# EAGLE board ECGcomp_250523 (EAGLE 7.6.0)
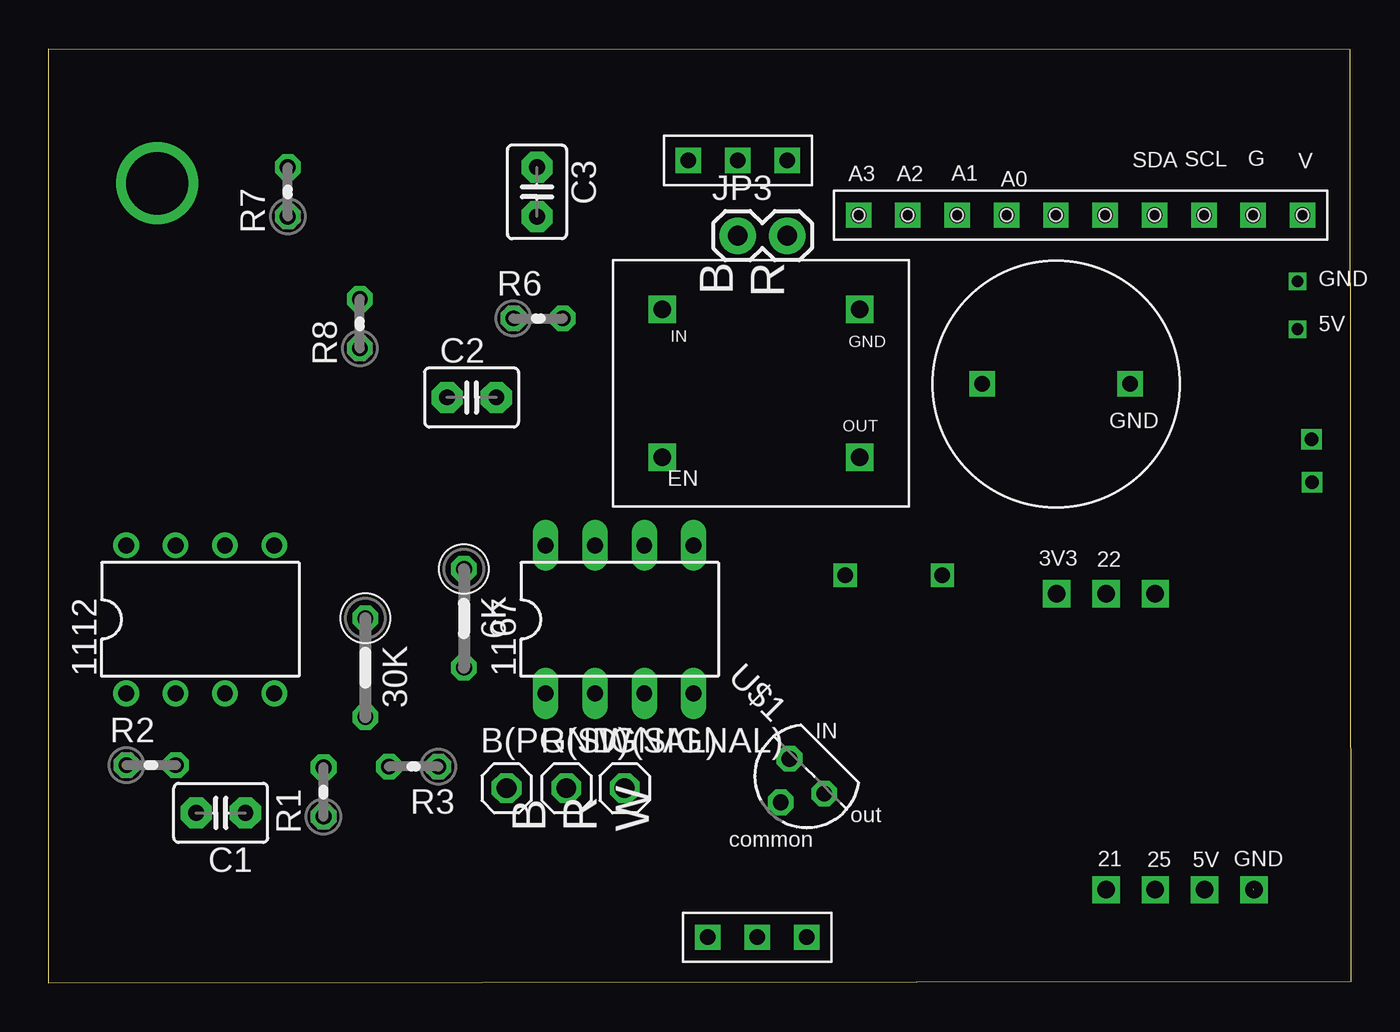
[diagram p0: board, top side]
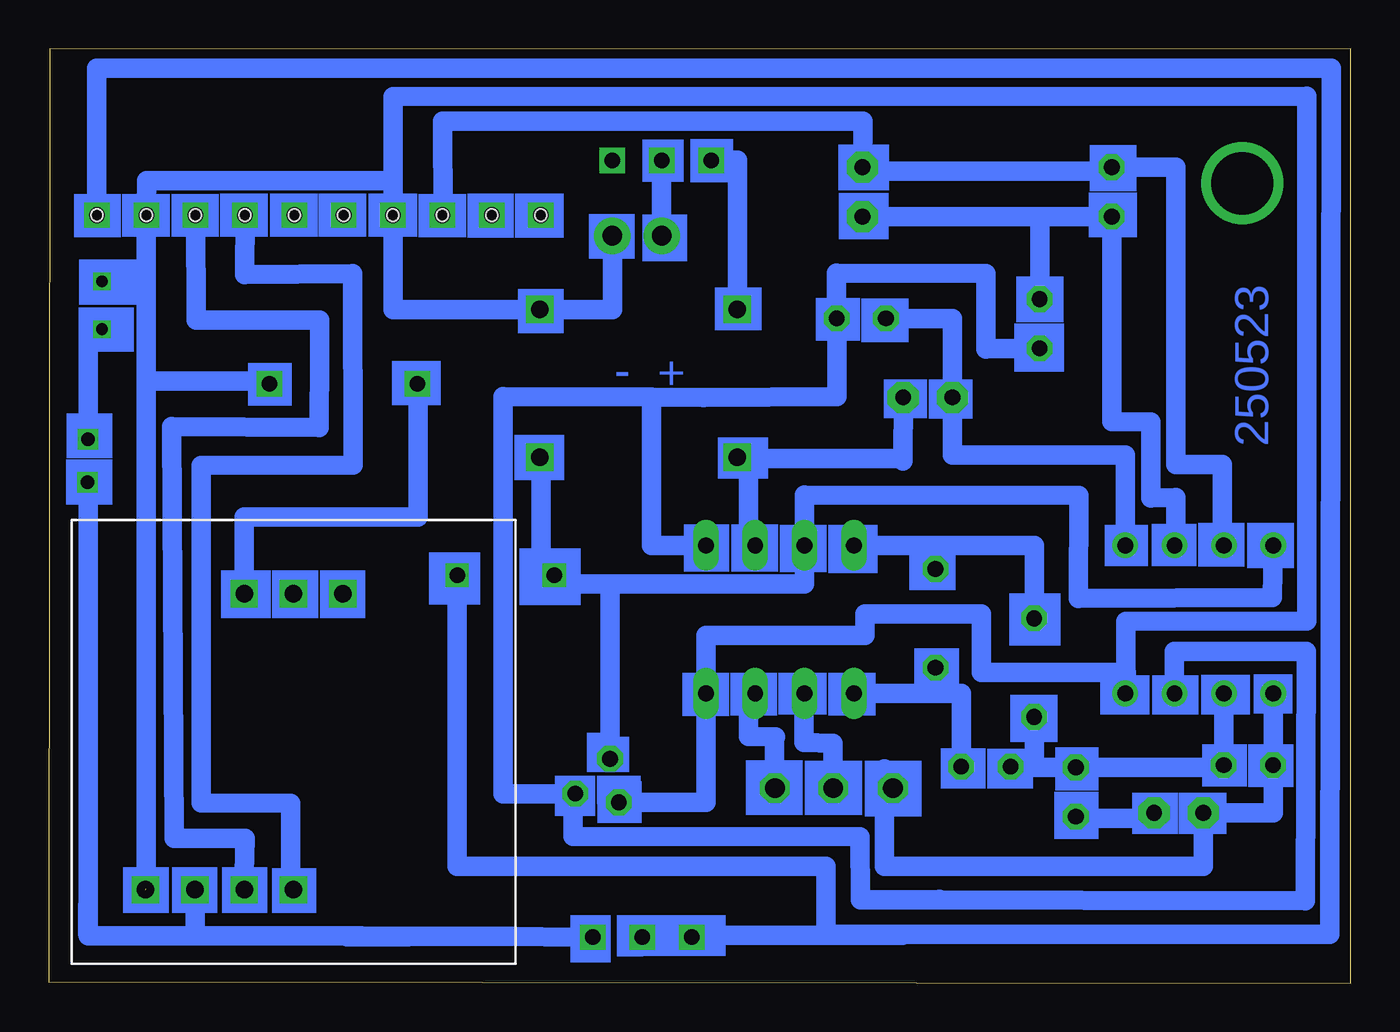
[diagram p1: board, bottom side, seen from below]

Size 67.03 x 48.1 mm. Coordinates in mm from the lower left corner, seen from the top.
Outline: 66.98,48.08 67.03,0.08 0,0 0,48.1 66.98,48.08
Copper layers (1*16): Top 0.035mm / dielectric 1.5mm / Bottom 0.035mm
Design rules "Fusion_eagle_rule_v1.1": minimum track width 6mil, minimum drill 12mil, track to track 6mil, track to pad 6mil, pad to pad 6mil, via to via 6mil, smd to smd 0mil, copper to edge 10mil, drill to drill 10mil, minimum pad ring 10mil, minimum via ring 6mil, stop-mask expansion 2mil, vias tented up to drill 100mil, thermal gap 10mil
Net classes: 0 default: width 1.016 mm

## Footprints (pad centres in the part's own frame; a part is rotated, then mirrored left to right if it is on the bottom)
0207/5V = drill 0.813 octagon: 1 -2.54,0; 2 2.54,0
DIL08 = drill 0.813 pad 1.27: 1 -3.81,-3.81; 2 -1.27,-3.81; 3 1.27,-3.81; 4 3.81,-3.81; 5 3.81,3.81; 6 1.27,3.81; 7 -1.27,3.81; 8 -3.81,3.81
DIL08' = drill 0.813 long: 1 -3.81,-3.81; 2 -1.27,-3.81; 3 1.27,-3.81; 4 3.81,-3.81; 5 3.81,3.81; 6 1.27,3.81; 7 -1.27,3.81; 8 -3.81,3.81
1X01 = drill 1.016 octagon: 1 0,0
C2.5-3 = drill 0.813 pad 1.6 octagon: 1 -1.27,0; 2 1.27,0
1X02 = drill 1.016 pad 1.88: 1 0,0; 2 2.54,0
0204V = drill 0.813 octagon: 1 -1.27,0; 2 1.27,0
TO226AA = drill 0.813 octagon: 1 -1.27,0; 2 0,1.905; 3 1.27,0
2 = drill 0.9 square: 3V3 -5.08,0; 5V 10.16,-7.62; G 10.16,-10.16; G19 -5.08,-5.08; G21 10.16,-2.54; G22 -5.08,-2.54; G25 10.16,-5.08
BUZZER = drill 0.8 square: LONG+ 2.54,0; SHORT- -5.08,0
SW1 = drill 0.8 square: SW1 -2.54,1.27; SW2 -5.08,1.27; SW3 -7.62,1.27
ADCHENGE2 = drill 0.8 square: 5V 7.62,5.08; A0 -7.62,5.08; A1 -10.16,5.08; A2 -12.7,5.08; A3 -15.24,5.08; ADDR -2.54,5.08; ALERT -5.08,5.08; GND 5.08,5.08; SCL 2.54,5.08; SDA 0,5.08 | hole 0.6: -15.24,5.08; -12.7,5.08; -10.16,5.08; 7.62,5.08; 5.08,5.08; 2.54,5.08; 0,5.08; -2.54,5.08; -5.08,5.08; -7.62,5.08
MCP1640 = drill 0.9 square: EN 2.54,-5.08; GND -5.08,5.08; VIN -5.08,-5.08; VOUT 2.54,5.08

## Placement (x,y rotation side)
6K  R5  [0207/5V]  21.37,18.78 270 top
30K  R4  [0207/5V]  16.29,16.24 270 top
1112  LT1112  [DIL08]  7.79,18.73 0 top
1167  LT1167CN8  [DIL08']  29.38,18.73 0 top
B(PGND)  [1X01]  23.56,10.03 0 top
C1  0.01uF  [C2.5-3]  8.85,8.76 180 top
C2  0.47uF  [C2.5-3]  21.76,30.16 0 top
C3  15nF  [C2.5-3]  25.13,40.74 270 top
JP3  Battery  [1X02]  35.47,38.48 0 top
R1  12k  [0204V]  14.14,9.84 90 top
R2  1M  [0204V]  5.26,11.22 0 top
R3  30k  [0204V]  18.78,11.15 180 top
R6  6k  [0204V]  25.19,34.22 0 top
R7  10k  [0204V]  12.3,40.74 90 top
R8  100k  [0204V]  16.01,33.95 90 top
R(SIGNAL)  [1X01]  26.64,10.03 0 top
U$1  TLE2426CLP  [TO226AA]  39.02,10.65 135 top
U$2  2  [2]  51.88,14.96 270 bottom
U$3  BUZZER  [BUZZER]  50.58,30.84 180 top
U$4  SW1  [SW1]  31.39,3.63 180 top
U$5  ADCHENGE2  [ADCHENGE2]  56.92,34.46 0 top
U$6  SW1  [SW1]  30.39,43.63 180 top
U$8  MCP1640  [MCP1640]  36.66,29.61 270 top
W(SIGNAL)  [1X01]  29.64,10.03 0 top

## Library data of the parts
6K 30K R1-R3 R6-R8 = resistor
1112 = linear
1167 = linear-technology; MPN: LT1168CN8#PBF; OC_FARNELL: 1330587; OC_NEWARK: 57M2327
B(PGND) R(SIGNAL) W(SIGNAL) = pinhead
C1-C3 = capacitor-wima
JP3 = SparkFun-Connectors
U$1 = tle2426
U$2 = M5Atom_Lite
U$3 = buzzer
U$4 U$6 = Switch1
U$5 = ADChenge
U$8 = MCP1640

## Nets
B1: 1112.3 1167.5 R6.2 R8.1 U$1.1
N$1: 1112.1 B(PGND).1 C1.2 R2.1
N$2: W(SIGNAL).1
N$3: 30K.2 1112.2 R1.2 R2.2 R3.2
N$4: 6K.2 1167.1 R3.1
N$5: 6K.1 30K.1 1167.8
N$6: 1167.2 R(SIGNAL).1
N$7: 1112.8 1167.7 U$1.3 U$8.VOUT
N$8: 1167.6 C2.2
N$9: 1112.5 C2.1 R6.1
N$10: 1112.6 C3.2 R7.1 R8.2
N$11: C1.1 R1.1
N$12: 1112.7 C3.1 R7.2 U$5.A1
N$13: 1112.4 1167.4 JP3.2 U$1.2 U$5.A0 U$8.GND
N$16: JP3.1 U$6.SW2
N$17: U$5.5V
N$18: U$2.G U$3.SHORT- U$5.GND
N$19: U$2.G25 U$5.SCL
N$20: U$2.G21 U$5.SDA
N$21: U$2.G19 U$3.LONG+
N$22: U$6.SW1 U$8.VIN
S$2: U$2.5V

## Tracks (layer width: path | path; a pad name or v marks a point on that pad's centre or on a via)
B1
  Bottom 1.016: 1112.3 9.08,14.92 9.08,17.08 2.29,17.08 2.34,4.24 25.24,4.29 | 40.01,9.66 U$1.1 | 18.78,32.68 18.78,36.53 26.46,36.56 R6.2 26.58,34.2 26.45,34.2 26.45,30.21 33.32,30.16 36,30.17 | U$1.1 43.65,9.75 43.65,30.21 36,30.17 | 36,30.17 36,22.54 1167.5 | R8.1 18.78,32.68 | 18.78,32.68 18.78,32.65 | U$1.1 40,9.75 40.02,7.56 25.27,7.53 25.24,4.29 | 25.24,4.29 21.18,4.31
N$1
  Bottom 1.016: 1112.1 3.99,14.92 R2.1 3.99,8.76 C1.2 7.58,6 24,6 24,11.03 B(PGND).1
N$2
  Bottom 1.016: 29.67,12.51 W(SIGNAL).1
N$3
  Bottom 1.016: 1112.2 6.53,14.92 R2.2 6.53,11.11 R1.2 16.29,11.11 | 16.29,11.11 17.51,11.11 R3.2 | 30K.2 16.29,11.11
N$4
  Bottom 1.016: 1167.1 25.41,14.92 21.37,14.92 | 21.37,14.92 20.05,14.92 R3.1 | 6K.2 21.37,14.92
N$5
  Bottom 1.016: 1167.8 21.37,22.54 | 21.37,22.54 16.29,22.54 30K.1 | 6K.1 21.37,22.54
N$6
  Bottom 1.016: 1167.2 28.15,14.92 28.15,12.38 26.64,12.34 R(SIGNAL).1
N$7
  Bottom 1.016: 1112.8 4.02,19.85 14.03,19.8 13.98,25.11 28.11,25.13 1167.7 28.11,20.56 38.12,20.56 | 38.12,20.56 U$1.3 | 38.12,20.56 41.69,20.56 41.69,27.07 U$8.VOUT
N$8
  Bottom 1.016: C2.2 23.05,26.88 23.05,27 31,27 31,22.54 1167.6
N$9
  Bottom 1.016: R6.1 20.49,34.22 C2.1 20.5,30.16 20.5,27.19 11.6,27.19 1112.5
N$10
  Bottom 1.016: C3.2 16,39.47 | 16,39.47 R7.1 12.3,28.91 10.29,28.89 10.29,24.98 9,25 9,22.54 1112.6 | R8.2 16,39.47
N$11
  Bottom 1.016: R1.1 13.72,8.49 10.22,8.49 C1.1
N$12
  Bottom 1.016: U$5.A1 46.72,39.54 46.74,44.38 25.1,44.38 C3.1 24.82,41.79 12.56,41.79 R7.2 9,42 9,26.7 6.61,26.7 6.61,22.54 1112.7
N$13
  Bottom 1.016: 11.39,14.92 1112.4 11.54,14.92 11.54,16 11.56,16 | U$1.2 33.19,9.3 1167.4 33.18,14.92 33.18,17.89 25,17.89 25,19 19,19 19,16 11.56,16 | 38.01,34.68 38.01,34.69 | 49.3,34.68 49.3,34.69 | 49.3,34.69 U$5.A0 49.3,45.64 2.27,45.67 2.27,18.65 11.56,18.63 11.56,16 | 38.01,34.69 U$8.GND 49.3,34.69 | 38.01,34.69 JP3.2
N$14  (via drill 0.6)
  other vias: 64.28,33.67
N$15  (via drill 0.6)
  other vias: 64.28,36.13
N$16
  Bottom 1.016: U$6.SW2 JP3.1
N$17
  Bottom 1.016: U$5.5V 64.57,39.54 64.57,47.1 1,47.1 1.08,2.5 27.08,2.5
N$18  (1 unrouted)
  Bottom 1.016: U$5.GND 62,31 | 62,31 55.66,31 U$3.SHORT- | 62.01,4.86 62.01,4.96 62.01,22.1 62,22 62,31
N$19
  Bottom 1.016: U$2.G25 57,4.8 56.92,7.46 60.56,7.46 60.69,28.66 53.12,28.61 53.09,32.32 53.09,34.15 59.44,34.15 U$5.SCL
N$20
  Bottom 1.016: U$2.G21 54.56,4.8 54.56,9.26 59.19,9.29 59.19,26.64 51.35,26.67 51.38,36.53 56.95,36.48 U$5.SDA
N$21
  Bottom 1.016: U$3.LONG+ 48,30.84 48,24 56.96,24 U$2.G19
N$22
  Bottom 1.016: U$6.SW1 31.58,42.36 U$8.VIN
N$23  (via drill 0.7)
  other vias: 65.02,25.79
N$24
  Bottom 1.016: 62,40 61.98,41.31 49.59,41.31
N$27  (via drill 0.8)
  other vias: 41,21
N$28  (via drill 0.7)
  Bottom 1.016: 64,34 65,34 v65,28
N$29  (via drill 3.2)
  other vias: 5.58,41.18
N$31  (via drill 0.8)
  Bottom 1.016: v46,21 46,6 27,6 27,3
N$32
  Bottom 1.016: 65,26 65,4 | 65,4 65,3 | 65,4 65.02,4 65.02,2.52
S$1
  Bottom 1.016: 29.62,12.67 31,12.7 31,15
S$2
  Bottom 1.016: U$2.5V 59.49,2.42 | 59.49,2.42 65,2.42 | 59.49,2.42 50.95,2.42 50.95,2.41
S$3
  Bottom 1.016: 48.51,2.39 51.66,2.39 51.66,2.41 43.06,2.41 40.06,2.36
S$4
  Bottom 1.016: 34.08,2.46 23.08,2.46
(copper drawn outside any net)
  shapes: Bottom area x92

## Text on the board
Bottom: + | - | 250523
tPlace: SDA | SCL | G | V | A3 | A2 | A1 | A0 | B / R | GND | 5V | IN | GND | GND | OUT | EN | 3V3 | 22 | IN | B / R / W | out | common | 21 | 25 | 5V | GND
